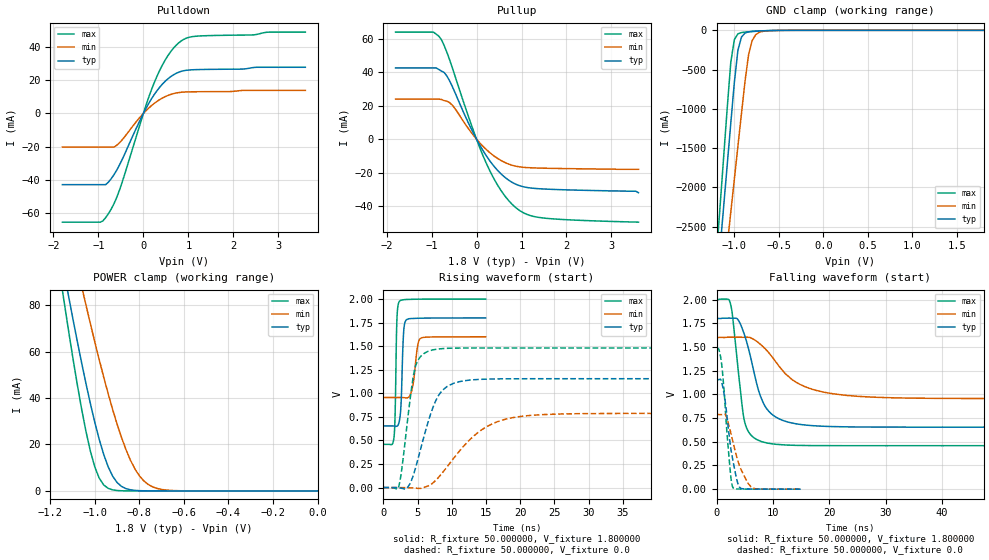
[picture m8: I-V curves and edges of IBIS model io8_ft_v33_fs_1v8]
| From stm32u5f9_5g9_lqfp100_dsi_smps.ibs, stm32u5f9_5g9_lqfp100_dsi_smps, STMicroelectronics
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|   Model io8_ft_v33_fs_1v8
[Model]  io8_ft_v33_fs_1v8
Model_type I/O
Polarity   Non-Inverting
Enable   Active-Low
Vinl =   0.540000V
Vinh =   1.260000V
Vmeas =  0.900000V
Cref =   50.000000pF
Rref =   100.000000M
Vref =   0.0V
C_comp   3.087500pF   3.086600pF   3.135700pF
[Temperature Range]   25.000000   0.140000k   -40.000000
[Pullup Reference]   1.800000V   1.600000V   2.000000V
[Pulldown Reference]   0.0V   0.0V   0.0V
[POWER Clamp Reference]   1.800000V   1.600000V   2.000000V
[GND Clamp Reference]   0.0V   0.0V   0.0V
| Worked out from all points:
|   slope of the pulldown table from 0 to 0.27 V, typ, clamps not added: 21.7 ohm
|   slope of the pullup table from 0 to 0.27 V, typ, clamps not added: 22.6 ohm
|   GND clamp passes 1 mA (typ) near -0.51 V on its own axis
|   POWER clamp passes 1 mA (typ) near -0.86 V on its own axis
|   rising waveform, R_fixture 50.000000, V_fixture 1.800000: 20-80 % time 317ps typ, 629ps min, 229ps max; typ from 0.654 V to 1.8 V
|   rising waveform, R_fixture 50.000000, V_fixture 0.0: 20-80 % time 2.89ns typ, 6.11ns min, 1.52ns max; typ from 0 V to 1.16 V
|   falling waveform, R_fixture 50.000000, V_fixture 1.800000: 20-80 % time 3.27ns typ, 6.78ns min, 1.71ns max; typ from 1.8 V to 0.654 V
|   falling waveform, R_fixture 50.000000, V_fixture 0.0: 20-80 % time 1.6ns typ, 2.38ns min, 1.14ns max; typ from 1.16 V to 0 V
[Pulldown]
|Voltage   I(typ)   I(min)   I(max)
-1.8V     -42.74mA   -20.21mA   -65.25mA
-960mV    -42.74mA   -20.21mA   -65.25mA
-780mV    -41.3mA    -20.21mA   -60.25mA
-660mV    -37mA      -20.2mA    -54.5mA
-540mV    -31.39mA   -17.82mA   -46.65mA
0V        -10fA      0A         10fA
240mV     11.28mA    6.002mA    18.38mA
480mV     19.18mA    10.02mA    31.83mA
780mV     24.67mA    12.5mA     42.21mA
960mV     25.9mA     12.9mA     45.21mA
1.14V     26.24mA    12.99mA    46.23mA
3.6V      27.69mA    13.82mA    48.79mA
[Pullup]
|Voltage   I(typ)   I(min)   I(max)
-1.8V     42.59mA    23.91mA    63.98mA
-960mV    42.59mA    23.91mA    63.98mA
-780mV    40.7mA     23.74mA    59.39mA
-660mV    37.78mA    22.66mA    52mA
-540mV    31.58mA    20.35mA    42.82mA
-120mV    6.338mA    4.065mA    8.965mA
180mV     -8.368mA   -5.234mA   -12.14mA
540mV     -20.62mA   -12.68mA   -30.5mA
900mV     -27.22mA   -16.28mA   -41.49mA
1.14V     -28.94mA   -17mA      -45.14mA
1.5V      -29.77mA   -17.34mA   -47.14mA
3.6V      -32mA      -18mA      -49.6mA
[GND_clamp]
|Voltage   I(typ)   I(min)   I(max)
-1.8V     -9.707A    -9.942A    -9.774A
-1.2V     -3.309A    -4.006A    -2.864A
-1.16V    -2.777A    -3.584A    -2.239A
-1.12V    -2.246A    -3.162A    -1.614A
-1.04V    -1.186A    -2.319A    -408.6mA
-1V       -663.9mA   -1.898A    -117.8mA
-960mV    -254mA     -1.478A    -45.14mA
-920mV    -86.03mA   -1.06A     -28.58mA
-840mV    -19.12mA   -308.9mA   -18.74mA
-800mV    -13.39mA   -130.8mA   -15.31mA
-720mV    -7.948mA   -25.37mA   -9.381mA
1.8V      0A         14.97nA    0A
[POWER_clamp]
|Voltage   I(typ)   I(min)   I(max)
-1.8V     470.8mA    433.7mA    554.6mA
-1.14V    95.25mA    122.7mA    82.82mA
-1.12V    84.97mA    114mA      70.27mA
-1.06V    55.51mA    88.42mA    35.67mA
-1.04V    46.34mA    80.15mA    25.76mA
-1V       29.51mA    64.13mA    10.3mA
-940mV    10.39mA    41.86mA    1.109mA
-900mV    3.624mA    28.77mA    182.8uA
-840mV    490.7uA    13.24mA    11.35uA
-800mV    116.8uA    6.532mA    1.77uA
-740mV    13.2uA     1.723mA    109.3nA
0V        0A         18.72nA    0A
[Ramp]
| variable   typ   min   max
dV/dt_r  0.69306/2.88612n   0.47206/6.10562n   0.88872/1.51791n
dV/dt_f  0.68762/3.26462n   0.38677/6.77012n   0.92481/1.71012n
R_load = 50.000000
[Rising Waveform]
R_fixture= 50.000000
V_fixture= 1.800000
V_fixture_min= 1.600000
V_fixture_max= 2.000000
|time   V(typ)   V(min)   V(max)
0s        654mV      955.4mV    458.7mV
1.562ns   653.4mV    955.4mV    541.2mV
1.712ns   652.2mV    955.4mV    779.4mV
1.982ns   650.8mV    955.4mV    1.792V
2.342ns   710.5mV    955.4mV    1.976V
2.583ns   885.5mV    955.2mV    1.988V
2.943ns   1.631V     954.3mV    1.993V
3.333ns   1.777V     951.4mV    1.995V
5.345ns   1.797V     1.578V     1.999V
14.95ns   1.8V       1.6V       2V
[Rising Waveform]
R_fixture= 50.000000
V_fixture= 0.0
V_fixture_min= 0.0
V_fixture_max= 0.0
|time   V(typ)   V(min)   V(max)
0s        4.575uV    -1.109uV   13.17uV
2.242ns   -3.065mV   5.751uV    10.23mV
3.524ns   3.052mV    -686.1uV   709.3mV
4.645ns   194.7mV    -6.054mV   1.274V
7.207ns   841.9mV    46.63mV    1.461V
8.649ns   1.033V     159.2mV    1.474V
10.25ns   1.106V     308.4mV    1.479V
14.41ns   1.149V     614.6mV    1.481V
19.86ns   1.154V     752.7mV    1.481V
79.76ns   1.155V     786.8mV    1.481V
[Falling Waveform]
R_fixture= 50.000000
V_fixture= 1.800000
V_fixture_min= 1.600000
V_fixture_max= 2.000000
|time   V(typ)   V(min)   V(max)
0s        1.8V       1.6V       2V
2.402ns   1.804V     1.603V     1.971V
2.883ns   1.803V     1.603V     1.807V
3.684ns   1.797V     1.603V     1.349V
4.965ns   1.627V     1.602V     715.9mV
8.008ns   950.4mV    1.516V     501.1mV
9.93ns    785mV      1.39V      477.7mV
13.61ns   695mV      1.147V     463.1mV
20.66ns   660.1mV    1.006V     459mV
79.76ns   654mV      955.4mV    458.7mV
[Falling Waveform]
R_fixture= 50.000000
V_fixture= 0.0
V_fixture_min= 0.0
V_fixture_max= 0.0
|time   V(typ)   V(min)   V(max)
0s        1.155V     786.8mV    1.481V
420.4ps   1.155V     786.8mV    1.472V
930.9ps   1.124V     786.6mV    1.308V
1.622ns   888.9mV    779.7mV    787.5mV
2.372ns   501.2mV    632.7mV    232.5mV
2.673ns   377.3mV    558.4mV    69.9mV
2.943ns   291.3mV    491mV      13.08mV
4.024ns   25.45mV    255.5mV    1.783mV
6.126ns   1.402mV    23.7mV     627.6uV
14.95ns   4.575uV    -1.109uV   13.17uV
